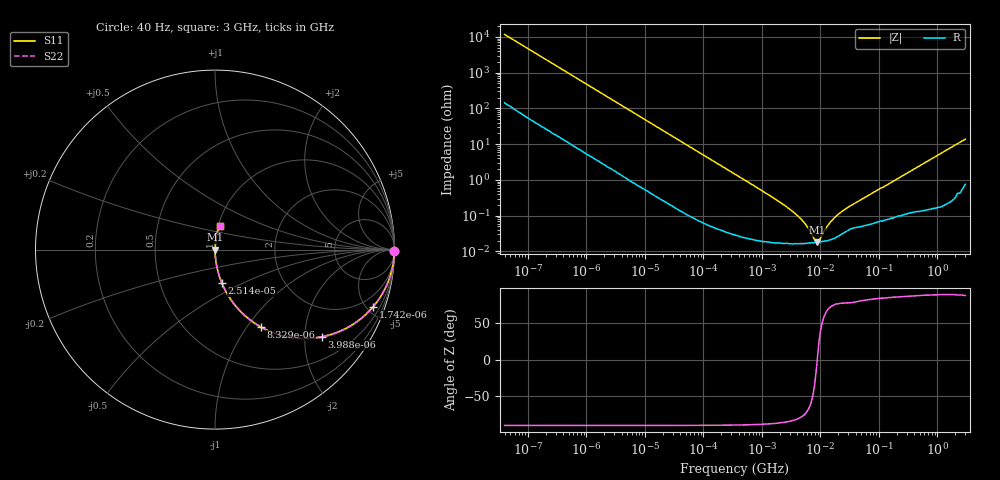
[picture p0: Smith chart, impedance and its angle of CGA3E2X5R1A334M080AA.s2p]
! S-parameter Generated by TDK Corporation
! Copyright(C) 2015 TDK Corporation.
! All Rights Reserved.
! TDK P/N: CGA3E2X5R1A334M080AA (Multilayer Ceramic Chip Capacitors)
! Property: C=330nF
! Size(LxWxT): 1.6x0.8x0.8mm, 0.063x0.031x0.031inches
! Model Type: s2p (Touchstone File Format Version 1.0)
! Frequency: DC=Yes Start=0.00004MHz Stop=3000MHz 396points Log-sweep
! Note: This model was converted from impedance.
! Model Generated on Jun. 23, 2015
! Hash(MD5):
! Port Assignments:
!  1 ---| |--- 2
! Applicable Conditions:
!  Temperature = 25 degC
!  DC Bias Voltage = 0 V
!  Small Signal Operation
! Terms and conditions regarding TDK Simulation Models
! (1)This simulation model is being provided solely for informational purposes. Please refer to the specifications of the products in terms of detailed characteristics of such products.
! (2)In no event shall TDK Corporation of any of its subsidiaries be liable for any loss or damage arising, directly or indirectly,
!  From any information contained in this simulation model, including, but not limited to loss or damages arising from any inaccuracies, omissions or errors in connection with such information.
! (3)Any and all copyrights on this simulation model are owned by TDK Corporation.
!  Duplication or redistribution of this simulation model without prior written permission from TDK Corporation is prohibited.
! (4)This simulation model is subject to any modification or change without any prior notice.
! (5)Neither TDK Corporation nor any of its subsidiaries shall make any warranty, express or implied,
!  Including but not limited to the correctness, implied warranties of merchantability and fitness for a particular purpose with respect to this simulation models.
! (6)The use of this simulation model shall be deemed to have consented to the terms and conditions hereof.
# MHz S MA R 50
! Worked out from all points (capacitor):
!   395 points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, 40 Hz to 3 GHz, reference 50 ohm
!   read as one part in series: C = 339 nF near 41.88 Hz
!   lowest |Z| = 18.1 mohm at 8.684 MHz (marker M1)
!   series resonance near 8.837 MHz, so ESL is about 960 pH
!   S11 on the Smith chart (normalised r, x): 40 Hz: open; 1.742 kHz: 1.06, -5.52; 3.988 kHz: 1.03, -2.42; 8.329 kHz: 1.01, -1.17; 25.14 kHz: 1.00, -0.39; 3 GHz: 1.02, +0.28
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4e-05  0.9999 -0.5  0.008536 88.8  0.008536 88.8  0.9999 -0.5
0.0002520917  0.998 -3.0  0.05296 86.3  0.05296 86.3  0.998 -3.0
0.000834128  0.9833 -9.9  0.1714 79.5  0.1714 79.5  0.9833 -9.9
0.001741936  0.9369 -19.8  0.3395 69.5  0.3395 69.5  0.9369 -19.8
0.003988472  0.7671 -39.3  0.6331 50.1  0.6331 50.1  0.7671 -39.3
0.008329251  0.5013 -59.3  0.8598 30.1  0.8598 30.1  0.5013 -59.3
0.01739424  0.2698 -73.7  0.96 15.7  0.96 15.7  0.2698 -73.7
0.02513652  0.1913 -78.3  0.9794 11.0  0.9794 11.0  0.1913 -78.3
0.0724464  0.06839 -85.4  0.9969 3.9  0.9969 3.9  0.06839 -85.4
0.3464102  0.01451 -88.0  0.9996 0.8  0.9996 0.8  0.01451 -88.0
3.154924  0.001415 -83.3  0.9998 0.1  0.9998 0.1  0.001415 -83.3
4.998775  0.000707 -76.4  0.9998 0.0  0.9998 0.0  0.000707 -76.4
7.22376  0.0002885 -52.6  0.9998 0.0  0.9998 0.0  0.0002885 -52.6
7.920238  0.0002136 -35.3  0.9998 0.0  0.9998 0.0  0.0002136 -35.3
8.683867  0.0001814 -6.7  0.9998 0.0  0.9998 0.0  0.0001814 -6.7
9.521122  0.0002053 26.4  0.9998 -0.0  0.9998 -0.0  0.0002053 26.4
13.75903  0.0005687 69.1  0.9998 -0.0  0.9998 -0.0  0.0005687 69.1
19.88326  0.001073 75.8  0.9997 -0.1  0.9997 -0.1  0.001073 75.8
31.50375  0.001831 76.9  0.9996 -0.1  0.9996 -0.1  0.001831 76.9
150.6385  0.007919 83.7  0.9992 -0.5  0.9992 -0.5  0.007919 83.7
906.6656  0.04405 85.4  0.9974 -2.5  0.9974 -2.5  0.04405 85.4
3000  0.1357 79.1  0.9833 -7.8  0.9833 -7.8  0.1357 79.1
